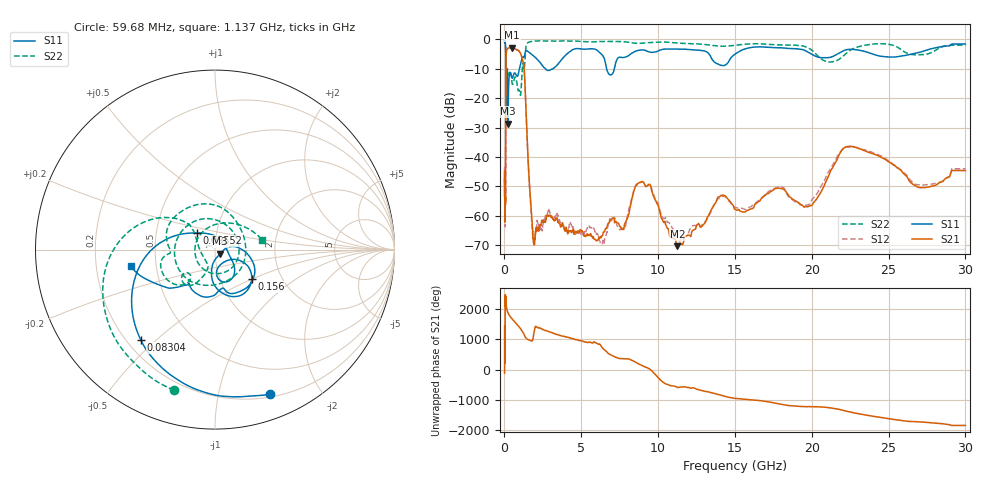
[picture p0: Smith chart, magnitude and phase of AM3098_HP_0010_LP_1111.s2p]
! Date/Time: Thu, Feb 28, 2019 8:33 AM
! Network Analyzer: Agilent Technologies E8364B Rev: A.07.50.67
! Sweep from 0.010 to 30.000 GHz, 1601 Points, Sweep Type: LOG
! Power Supply: 5.022 V, 0.002 A
# Hz S DB R 50
!freq MagS11 AngS11 MagS21 AngS21 MagS12 AngS12 MagS22 AngS22
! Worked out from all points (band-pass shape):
!   1601 points, 10 MHz to 30 GHz, reference 50 ohm
!   highest |S21| = -2.76 dB at 498 MHz (marker M1); lowest = -70.4 dB at 11.25 GHz (marker M2)
!   |S21| within 3 dB of the highest: 107.7 MHz to 1.113 GHz (1.006 GHz wide, 165 % of centre)
!   lowest |S11| = -28.6 dB at 232.8 MHz (marker M3), VSWR 1.08, Z = 52.9 - j2.49 ohm
!   |S11| at or under -10 dB: 92.13 MHz to 973 MHz (880.9 MHz wide, 165 % of centre); 2.668 GHz to 3.147 GHz (478.5 MHz wide, 16.5 % of centre); 6.649 GHz to 7.152 GHz (502.4 MHz wide, 7.28 % of centre)
!   |S22| runs from -22.4 to -0.5 dB; largest |S21 - S12| = 0.011
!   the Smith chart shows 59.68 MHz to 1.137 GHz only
!   S11 on the Smith chart (normalised r, x): 59.68 MHz: 0.23, -1.42; 83.04 MHz: 0.26, -0.45; 95.52 MHz: 0.81, +0.15; 156 MHz: 1.41, -0.49; 1.137 GHz: 0.36, -0.09
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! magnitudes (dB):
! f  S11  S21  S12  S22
! 10 MHz  -0.3  -47.5  -44.6  -0.6
! 38.04 MHz  -0.5  -61.7  -63.0  -1.1
! 48.37 MHz  -0.8  -51.6  -47.5  -1.4
! 59.68 MHz  -1.3  -54.1  -53.3  -1.8
! 74.38 MHz  -2.2  -50.5  -51.4  -2.6
! 83.04 MHz  -3.7  -34.4  -34.9  -4.1
! 95.52 MHz  -17.4  -11.6  -11.6  -20.6
! 144.7 MHz  -14.9  -3.5  -3.5  -13.0
! 156 MHz  -11.6  -3.5  -3.4  -11.1
! 232.8 MHz  -28.6  -2.9  -2.9  -11.9
! 498 MHz  -13.2  -2.8  -2.7  -14.9
! 550.5 MHz  -12.6  -2.9  -2.9  -15.1
! 1.137 GHz  -6.4  -6.2  -6.2  -11.4
! 1.302 GHz  -5.5  -11.5  -11.5  -9.2
! 1.866 GHz  -5.5  -67.6  -65.4  -0.6
! 2.084 GHz  -6.5  -64.7  -64.2  -0.5
! 7.926 GHz  -5.9  -61.8  -62.4  -0.8
! 9.164 GHz  -3.7  -49.8  -50.0  -1.1
! 11.25 GHz  -3.3  -70.4  -67.9  -1.2
! 19.8 GHz  -4.5  -56.8  -56.2  -3.0
! 22.67 GHz  -3.4  -36.5  -36.6  -3.2
! 30 GHz  -1.5  -44.6  -44.0  -1.9
